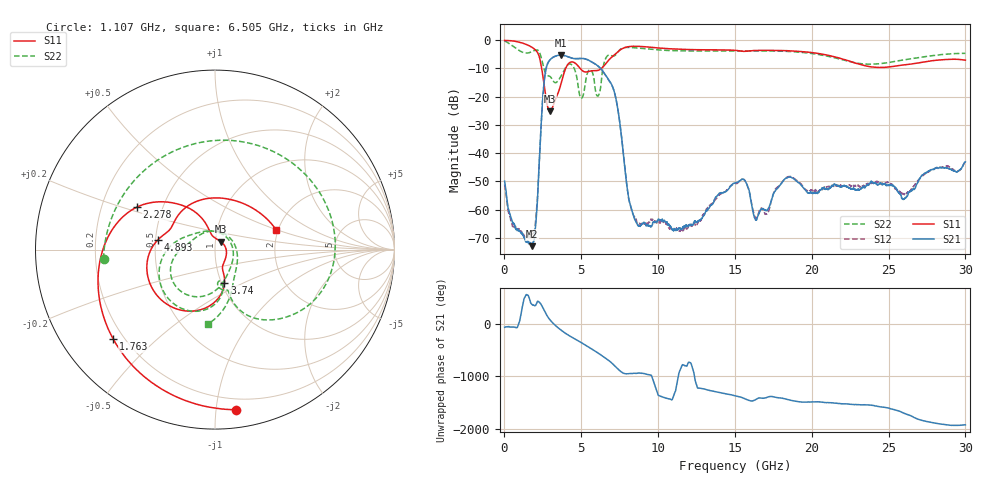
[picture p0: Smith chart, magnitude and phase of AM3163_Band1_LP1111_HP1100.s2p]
!Agilent Technologies,E8364B,MY43040894,A.07.50.67
!Agilent E8364B: A.07.50.67
!Date: Thursday, August 20, 2020 11:59:25
!Correction: S11(Full 2 Port(1,2))
!S21(Full 2 Port(1,2))
!S12(Full 2 Port(1,2))
!S22(Full 2 Port(1,2))
!S2P File: Measurements: S11, S21, S12, S22:
# Hz S  dB  R 50
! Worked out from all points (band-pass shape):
!   3201 points, 10 MHz to 30 GHz, reference 50 ohm
!   highest |S21| = -5.30 dB at 3.665 GHz (marker M1); lowest = -73.0 dB at 1.772 GHz (marker M2)
!   |S21| within 3 dB of the highest: 2.81 GHz to 5.864 GHz (3.054 GHz wide, 70.4 % of centre)
!   lowest |S11| = -25.2 dB at 2.953 GHz (marker M3), VSWR 1.12, Z = 53.1 + j4.73 ohm
!   |S11| at or under -10 dB: 2.422 GHz to 3.985 GHz (1.563 GHz wide, 48.8 % of centre); 4.927 GHz to 6.318 GHz (1.391 GHz wide, 24.7 % of centre)
!   |S22| runs from -20.5 to -0.3 dB; largest |S21 - S12| = 0.0052
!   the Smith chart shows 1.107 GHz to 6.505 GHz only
!   S11 on the Smith chart (normalised r, x): 1.107 GHz: 0.12, -1.13; 1.763 GHz: 0.16, -0.37; 2.278 GHz: 0.36, +0.22; 3.74 GHz: 1.03, -0.40; 4.893 GHz: 0.51, +0.06; 6.505 GHz: 1.95, +0.49
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1e7  -0.11 -5.2  -49.91 -59.2  -51.10 60.2  -0.34 -11.9
5.34825e8  -0.27 -39.4  -64.66 -56.7  -65.77 -56.8  -2.02 -86.7
1.106509e9  -0.92 -82.7  -68.52 -126.5  -67.80 150.2  -4.11 -175.2
1.762541e9  -2.44 -138.6  -72.73 25.0  -68.87 -179.5  -4.14 74.3
1.771912e9  -2.47 -139.5  -72.96 24.1  -68.86 -175.9  -4.11 72.6
2.277994e9  -6.11 151.3  -41.88 60.8  -42.33 65.2  -4.30 -29.9
2.952769e9  -25.24 54.3  -7.03 86.5  -7.05 86.5  -12.81 -78.2
3.665031e9  -15.78 -71.3  -5.30 -109.8  -5.32 -109.8  -12.90 -78.9
3.740006e9  -14.26 -74.2  -5.31 -126.4  -5.33 -126.3  -12.17 -80.8
4.892747e9  -9.78 170.7  -6.51 25.4  -6.48 25.3  -19.42 103.6
5.014581e9  -10.51 164.1  -6.48 4.2  -6.46 4.1  -20.54 42.2
6.504709e9  -8.92 18.0  -11.77 83.3  -11.85 83.3  -7.66 -95.0
7.5075e9  -3.55 -101.1  -29.23 -172.4  -29.22 -171.2  -3.41 -169.6
8.444688e9  -2.16 -176.4  -63.04 139.0  -62.57 132.0  -2.68 132.9
1.000979e10  -2.76 100.5  -63.39 77.1  -64.41 68.3  -3.45 65.6
1.227778e10  -3.36 9.7  -65.37 -156.5  -64.95 -123.3  -3.84 -15.0
1.5005e10  -3.59 -74.1  -50.56 67.2  -50.97 68.3  -3.78 -92.4
1.636392e10  -3.64 -104.5  -63.70 -2.9  -62.94 9.0  -3.79 -125.6
2.000958e10  -4.40 162.3  -53.96 -49.8  -53.15 -49.0  -4.72 135.7
2.274617e10  -7.97 59.7  -52.47 -99.8  -51.50 -95.7  -7.93 20.1
2.500479e10  -9.53 -63.1  -51.30 -167.3  -50.51 -170.3  -7.94 -93.1
3e10  -7.07 103.5  -43.10 -128.9  -42.72 -129.1  -4.67 100.8
